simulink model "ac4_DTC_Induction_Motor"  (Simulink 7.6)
settings: Solver=FixedStepDiscrete  StartTime=0.0  StopTime=6  FixedStep=Ts  RelTol=1e-3
InitFcn:
  | Ts=1e-5;
StopFcn:
  | close all
  | load Csg_Vit.mat
  | plot(x(1,:),x(2,:),x(1,:),x(3,:))
  | title('Consigne vitesse et vitesse de rotation')
  | xlabel('temps')
  | grid
  | 
  | figure
  | load I_w.mat
  | plot(y(1,:),y(2,:),y(1,:),y(3,:))
  | title('Courant stator (Phase A) et couple éléctromagnétique')
  | xlabel('temps')
  | grid
libraries: powerlib x2, electricdrivelib x1

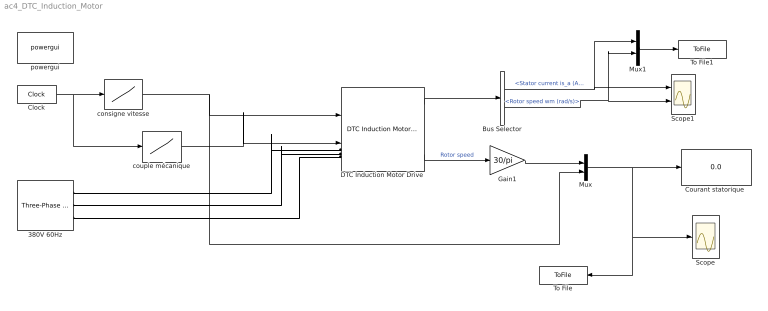
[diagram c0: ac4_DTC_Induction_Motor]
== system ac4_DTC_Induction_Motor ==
  380V 60Hz : powerlib/Electrical Sources/Three-Phase Source  DialogController=POWERSYS.PowerSysDialog  SystemSampleTime=-1  Voltage=380  PhaseAngle=0  Frequency=60  InternalConnection=Yg  SpecifyImpedance=off  Resistance=0.02  Inductance=0.05e-3  ShortCircuitLevel=100e6  BaseVoltage=25e3  XRratio=7
  Bus Selector : BusSelector  OutputSignals=Stator current is_a (A),Rotor speed wm (rad/s)
  Clock : Clock
  "Courant statorique " : Display
  DTC Induction Motor Drive : electricdrivelib/AC drives/DTC Induction Motor Drive  SystemSampleTime=-1  showMaskWarnings=on  AverageValue=off  MechanicalLoad=Torque Tm  driveType=AC4
  Gain1 : Gain  Gain=30/pi
  Mux : Mux  Inputs=2
  Mux1 : Mux  Inputs=2
  Scope : Scope
  Scope1 : Scope  NumInputPorts=2
  To File : ToFile  Filename=Csg_Vit  MatrixName=x
  To File1 : ToFile  Filename=I_w  MatrixName=y
  consigne vitesse : Lookup  InputValues=[0 0.25 2 4 5 6]  Table=[0 0 200 200 50 50]
  couple mécanique : Lookup  InputValues=[0 0.5 0.501 1.75 1.7501 2.25 2.2501 5]  Table=[0 0 -1000 -1000 -1000 -1000 1000 1000]
  powergui : powerlib/powergui  Priority=2  SystemSampleTime=-1  SimulationMode=Discrete  SampleTime=Ts  frequency=60  SPID=off  DisableSnubberDevices=off  DisableRonSwitches=off  DisableVfSwitches=off  SwTol=0  Interpol=off  frequencyindice=60  echomessages=off  HookPort=off  DisplayEquations=off  FunctionMessages=off  EnableUseOfTLC=off  x0status=blocks  RestoreLinks=warning  ResistiveCurrentMeasurement=off  Frange=[0:2:500]  Ylog=off  Xlog=on  ShowGrid=off  save=off  variable=ZData  ZoomFFT=on  StartTime=0.0  cycles=1  DisplayStyle=1  fundamental=60  FreqAxis=off  MaxFrequency=1000  frequencyindicesteady=1  RmsSteady=1  display=off  Ts=0  methode=off
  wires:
  couple mécanique/1 -> DTC Induction Motor Drive/2
  consigne vitesse/1 -> Mux/2, DTC Induction Motor Drive/1
  Clock/1 -> couple mécanique/1, consigne vitesse/1
  Mux/1 -> "Courant statorique "/1, Scope/1, To File/1
  DTC Induction Motor Drive/1 -> Bus Selector/1
  Gain1/1 -> Mux/1
  Mux1/1 -> To File1/1
  Bus Selector/1 -> Scope1/1, Mux1/1  "<Stator current is_a (A)>"
  Bus Selector/2 -> Scope1/2, Mux1/2  "<Rotor speed wm (rad/s)>"
  DTC Induction Motor Drive/4 -> Gain1/1  "Rotor speed"
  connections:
  380V 60Hz/RConn1 -- DTC Induction Motor Drive/LConn1
  380V 60Hz/RConn2 -- DTC Induction Motor Drive/LConn2
  380V 60Hz/RConn3 -- DTC Induction Motor Drive/LConn3
